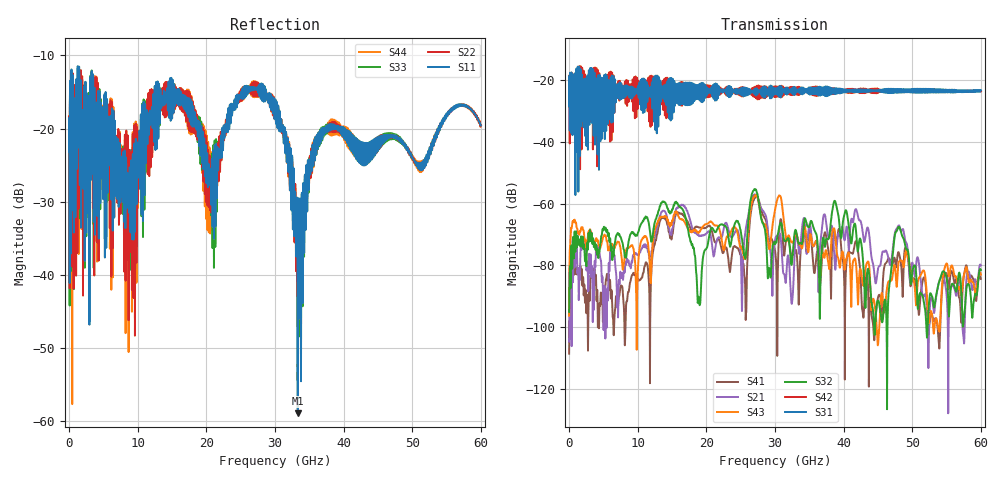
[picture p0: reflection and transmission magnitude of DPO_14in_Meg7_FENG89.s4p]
! Tyco Electronics Strada Whisper System
! FEXT_G89_G1112
!! SYSTEM DESCRIPTION: Daughtercard-Footprint-Connector-Footprint-Daughtercard
!! PCB DESCRIPTION: DC: 140mil, Megtron7N, upper layer route, 15mil stub, 6-6-6mil 14" traces
!! CONNECTOR DESCRIPTION: Next-Gen STRADA Whisper Direct-Plug Orthogonal Connector
!! MODEL DESCRIPTION: Tyco Electronics System 4-port S-parameter
!! MODEL STATUS: Developmental
!! MODEL GEOMETRY: Channel Model
!! MODEL FREQUENCY RANGE: DC to 60 GHz in 10 MHz frequency steps
!! MODEL EDGE RATE LIMITATION: 8.3 ps (Using conservative 0.5/Fmax rule of thumb)
!! TIME-DOMAIN TRANSFORM CAUTIONS:
!! 1.) Do not simulate transient edge rates faster than the number listed above.  Edge rates faster than this number
!!  contain significant spectral content at frequencies above the model's highest frequency.
!! 2.) Even when simulating edge rates that are slower than the number listed above, be aware that the best time
!!  resolution possible with a direct iFFT is (1 / 2Fmax).  As a result, time resolution is typically not adequate
!!  for most time-domain simulations unless tricks such as windowing are used to minimize leakage and aliasing.
!! 3.) Because the model has a uniform frequency step, a direct iFFT will result in an impulse that that has a time
!!  length given by either (1 / Fstep) or (1 / 2Fstep), depending on the transform being used.  Care has been taken
!!  in selecting the frequency step to ensure a settled impulse response for the model.  Therefore, convolution with
!!  the model's impulse response should present no issues.  However, if directly concatenating s-parameter models
!!  in the frequency domain a user must either interpolate necessary interim frequencies or complete impulse response
!!  zero-padding.  Impulse response zero-padding is more difficult, but more accurate.
!! PORT DEFINITIONS:
!! Port  1  ----->  TX Side	G8  G11  RX Side  <-----  Port  3
!! Port  2  ----->  TX Side	G9  G12  RX Side  <-----  Port  4
! Touchstone data
! Created: 10-Dec-2018 by IdEM R2012 (8.0.5)
# Hz S MA R 50
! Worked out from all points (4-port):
!   6000 points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, 10 MHz to 60 GHz, reference 50 ohm
!   strongest paths, dB at 10 MHz, 15.01 GHz, 30.01 GHz, 45.01 GHz, 60 GHz:
!     S31: -28.4, -30.5, -23.0, -23.2, -23.2
!     S42: -28.4, -27.1, -23.5, -24.1, -23.6
!     S32: -95.1, -61.8, -73.1, -91.4, -81.5
!     S43: -96.3, -65.4, -61.9, -105.8, -83.0
!     S21: -104.6, -68.2, -71.7, -81.1, -80.0
!     S41: -108.6, -70.0, -75.1, -90.5, -84.4
!   lowest |S11| = -59.0 dB at 33.32 GHz (marker M1), VSWR 1.00, Z = 50 - j0.105 ohm
!   |S11| at or under -10 dB: start of sweep to end of sweep
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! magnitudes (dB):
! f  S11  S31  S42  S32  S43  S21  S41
! 10 MHz  -23.2  -28.4  -28.4  -95.1  -96.3  -104.6  -108.6
! 13.71 GHz  -16.7  -23.7  -24.4  -59.4  -64.3  -62.3  -64.4
! 25.67 GHz  -14.3  -22.5  -23.3  -77.8  -78.0  -69.5  -87.9
! 27.26 GHz  -14.6  -24.7  -24.8  -55.6  -57.2  -57.1  -57.4
! 29.16 GHz  -15.1  -22.0  -24.3  -80.9  -74.8  -72.9  -72.1
! 33.32 GHz  -59.0  -23.7  -24.6  -71.9  -71.5  -72.2  -81.5
! 60 GHz  -19.6  -23.2  -23.6  -81.5  -83.0  -80.0  -84.4
